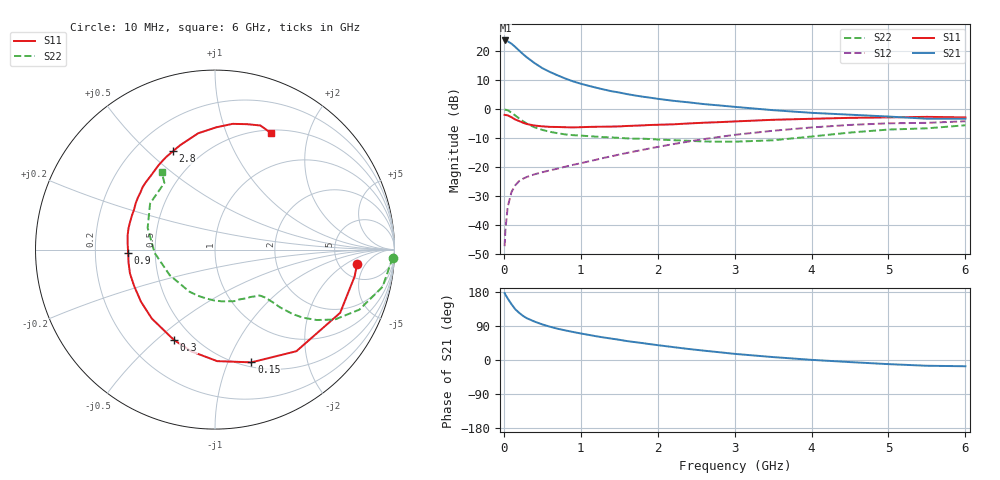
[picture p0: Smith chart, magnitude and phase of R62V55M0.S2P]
! SIEMENS Small Signal Semiconductors
! BFR193
! Si NPN RF Bipolar Junction Transistor in SOT23
! VCE = 2.5 V  IC = 5 mA
! Common Emitter S-Parameters:  May  1996
# GHz  S  MA  R  50
!  f  S11  S21  S12  S22
! GHz  MAG  ANG  MAG  ANG  MAG  ANG  MAG  ANG
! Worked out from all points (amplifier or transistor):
!   36 points, 10 MHz to 6 GHz, reference 50 ohm
!   highest |S21| = 23.7 dB at 20 MHz (marker M1)
!   |S21| within 3 dB of that: start of sweep to 179 MHz
!   unconditionally stable (mu >= 1): 879.5 MHz to 2.015 GHz
!   at 250 MHz: K = 0.43, MSG = 21.5 dB, |S12| = -24.0 dB
!   at 1.4 GHz: K = 1.07, MAG = 9.6 dB, |S12| = -16.3 dB
!   at 6 GHz: K = 0.97, MSG = 0.4 dB, |S12| = -4.2 dB
!   lowest NFmin = 1.20 dB at 450 MHz
!   S11 on the Smith chart (normalised r, x): 10 MHz: 7.41, -3.20; 150 MHz: 0.55, -1.22; 300 MHz: 0.39, -0.57; 900 MHz: 0.35, -0.02; 2.8 GHz: 0.35, +0.60; 6 GHz: 0.54, +1.45
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0.01  0.7961 -5.7  15.24 176.6  0.0043 87.8  0.991 -2.6
0.02  0.792 -11.0  15.36 172.6  0.008 84.7  0.9792 -5.1
0.05  0.7812 -26.8  14.86 162.4  0.0205 76.5  0.9566 -12.5
0.1  0.7254 -51.3  13.49 147.1  0.0372 66.3  0.8711 -22.6
0.15  0.6601 -72.1  11.82 133.6  0.0488 57.6  0.7726 -30.3
0.2  0.6215 -88.9  10.24 124.3  0.0574 52.9  0.6891 -34.7
0.25  0.5818 -103.2  8.902 116.3  0.0629 49.5  0.6184 -37.8
0.3  0.5525 -114.6  7.841 110.1  0.0676 47.9  0.5614 -39.7
0.4  0.5211 -132.5  6.238 101.3  0.075 46.7  0.4851 -41.6
0.5  0.5044 -144.9  5.114 93.9  0.0814 46.9  0.4383 -42.3
0.6  0.4941 -155.8  4.384 87.8  0.0877 48.4  0.406 -43.1
0.7  0.4921 -164.3  3.83 82.5  0.0941 49.9  0.3835 -43.9
0.9  0.4842 -177.8  3.017 73.9  0.1092 53.0  0.3556 -46.0
1.1  0.4931 171.0  2.535 66.4  0.1252 55.6  0.342 -49.7
1.3  0.4977 161.7  2.183 59.4  0.144 57.3  0.3288 -53.6
1.6  0.5122 149.5  1.821 50.0  0.1752 58.6  0.313 -61.7
2.2  0.5468 130.2  1.396 34.1  0.2488 56.6  0.2915 -81.8
2.8  0.5965 113.0  1.16 20.5  0.331 50.3  0.2744 -110.2
3.5  0.655 98.2  0.96 7.7  0.4237 39.5  0.2897 -150.5
4.5  0.7075 82.0  0.802 -5.5  0.5342 22.8  0.3943 162.1
5.5  0.7363 69.9  0.684 -15.2  0.5803 5.7  0.4664 127.2
6  0.7199 64.2  0.685 -16.5  0.6179 0.7  0.5269 124.4
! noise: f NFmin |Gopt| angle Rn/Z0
0.45  1.2  0.26  102  0.14
0.9  1.25  0.38  145  0.12
1.8  2.05  0.56  -161  0.12
